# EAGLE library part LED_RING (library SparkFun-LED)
Top Up Industry Corp 16 LED Ring - LED-CCLA 16 LEDs broken into quarters. 4 anode pins + 1 common ground / quadrant. Forward Voltage: Red 2.4V; Blue 3.0V Forward Current: Red 25mA; Blue 30mA Wavelength: Red 624nm; Blue 465nm SparkFun Products: Blue LED Ring Red LED Ring
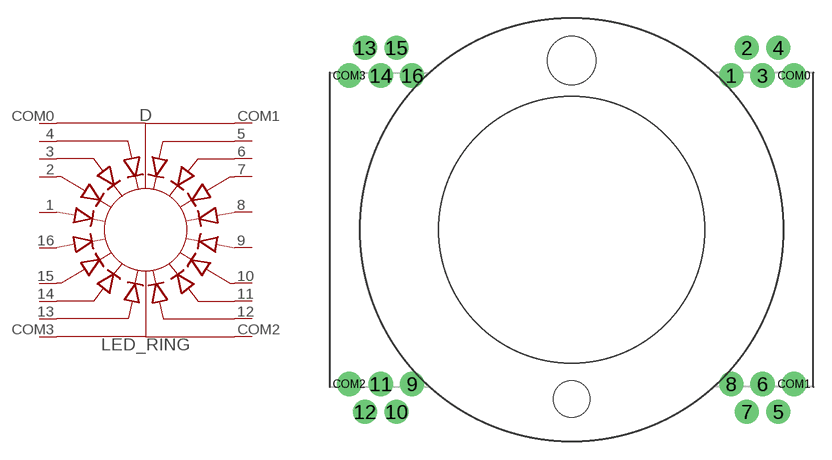
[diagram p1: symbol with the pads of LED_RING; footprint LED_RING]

Designator prefix D

## LED_RING (SF_ID: COM-10595)  [LED_RING]
1  1  pas
2  2  pas
3  3  pas
4  4  pas
5  5  pas
6  6  pas
7  7  pas
8  8  pas
9  9  pas
10  10  pas
11  11  pas
12  12  pas
13  13  pas
14  14  pas
15  15  pas
16  16  pas
COM0  COM0  pas
COM1  COM1  pas
COM2  COM2  pas
COM3  COM3  pas

## Footprint LED_RING (pad centres in mm)
16 LED Ring - LED-CCL-A Specifications: Pin count: 20 Area: 26 x 40mm Datasheet referenced for footprint: LED-CCL-A Example device(s): LED Ring
drill 1.2 pad 2: 1 13.2,12.75; 2 14.5,15.05; 3 15.8,12.75; 4 17.1,15.05; 5 17.1,-15.05; 6 15.8,-12.75; 7 14.5,-15.05; 8 13.2,-12.75; 9 -13.2,-12.75; 10 -14.5,-15.05; 11 -15.8,-12.75; 12 -17.1,-15.05; 13 -17.1,15.05; 14 -15.8,12.75; 15 -14.5,15.05; 16 -13.2,12.75; COM0 18.4,12.75; COM1 18.4,-12.75; COM2 -18.4,-12.75; COM3 -18.4,12.75
hole 4 at 0,14
hole 3 at 0,-14

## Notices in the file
Licensing: Creative Commons ShareAlike 4.0 International - https://creativecommons.org/licenses/by-sa/4.0
